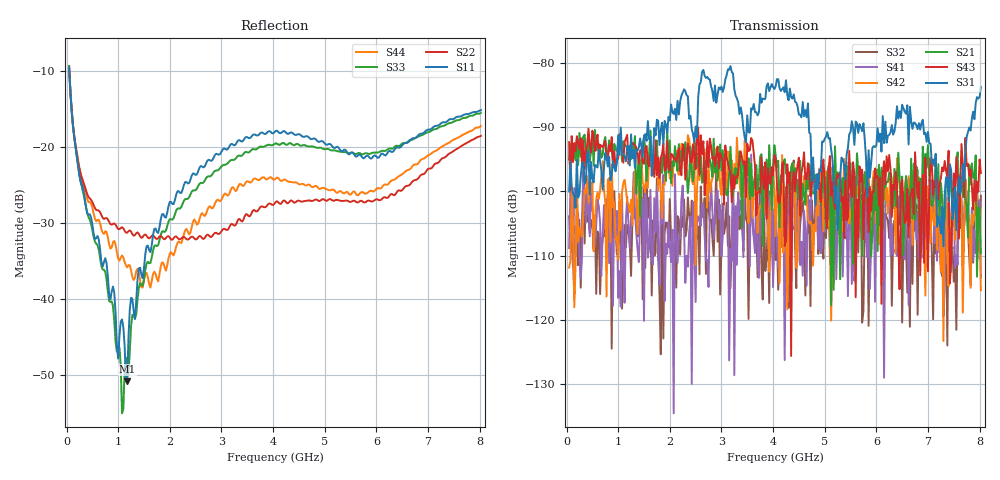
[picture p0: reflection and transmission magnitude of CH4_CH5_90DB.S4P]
!Agilent Technologies,E5071C,MY46316741,A.11.02
!Date: Mon Jun 01 11:45:32 2026
!Data & Calibration Information:
!1:CH4 INPUT 2:CH4 OUTPUT 3:CH5 INPUT 4:CH5 OUTPUT
!Freq	S11:SOLT4(ON)	S12:SOLT4(ON)	S13:SOLT4(ON)	S14:SOLT4(ON)
!	S21:SOLT4(ON)	S22:SOLT4(ON)	S23:SOLT4(ON)	S24:SOLT4(ON)
!	S31:SOLT4(ON)	S32:SOLT4(ON)	S33:SOLT4(ON)	S34:SOLT4(ON)
!	S41:SOLT4(ON)	S42:SOLT4(ON)	S43:SOLT4(ON)	S44:SOLT4(ON)
!PortZ  Port1:50+j0  Port2:50+j0  Port3:50+j0  Port4:50+j0
!Above PortZ is port z conversion or system Z0 setting when saving the data.
!When reading, reference impedance value at option line is always used.
# Hz S dB R 50
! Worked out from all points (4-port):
!   320 points, 50 MHz to 8.025 GHz, reference 50 ohm
!   strongest paths, dB at 50 MHz, 2.05 GHz, 4.05 GHz, 6.05 GHz, 8.025 GHz:
!     S31: -100.1, -87.7, -83.7, -92.3, -83.8
!     S43: -92.4, -94.3, -94.9, -102.2, -97.2
!     S21: -95.1, -95.4, -94.4, -95.9, -109.7
!     S42: -111.9, -99.2, -107.0, -108.1, -115.4
!     S41: -108.8, -106.0, -102.4, -102.6, -113.4
!     S32: -103.9, -108.2, -110.7, -108.1, -100.7
!   lowest |S11| = -50.9 dB at 1.175 GHz (marker M1), VSWR 1.01, Z = 49.8 - j0.208 ohm
!   |S11| at or under -10 dB: 53.71 MHz to end of sweep
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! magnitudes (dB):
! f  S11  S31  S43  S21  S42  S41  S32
! 50 MHz  -9.5  -100.1  -92.4  -95.1  -111.9  -108.8  -103.9
! 400 MHz  -28.7  -94.2  -92.7  -94.5  -97.7  -99.2  -104.7
! 1.075 GHz  -42.7  -94.1  -93.5  -95.4  -100.1  -100.8  -118.3
! 1.175 GHz  -50.9  -93.0  -91.2  -93.1  -101.7  -100.8  -105.3
! 1.55 GHz  -33.1  -92.2  -93.0  -98.4  -95.3  -101.6  -98.7
! 2.75 GHz  -21.7  -82.5  -96.3  -94.6  -95.7  -114.9  -102.7
! 8.025 GHz  -15.1  -83.8  -97.2  -109.7  -115.4  -113.4  -100.7
